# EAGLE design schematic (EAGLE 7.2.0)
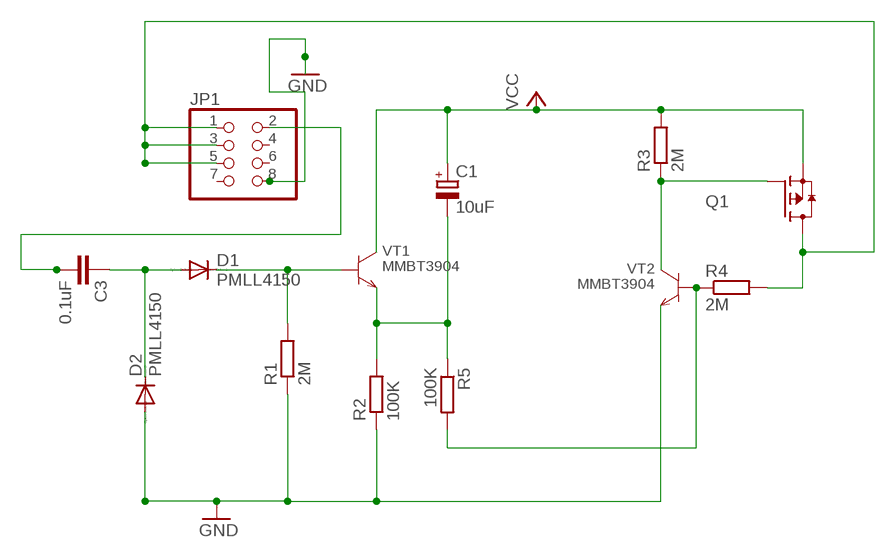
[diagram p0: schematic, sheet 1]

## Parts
C1  10uF  CPOL-EU153CLV-0505  [153CLV-0505]
C3  0.1uF  C-EUC0805  [C0805]
D1  PMLL4150  [SOD80C]
D2  PMLL4150  [SOD80C]
JP1  PINHD-2X4  [2X04]
Q1  BSS84  [SOT-23]
R1  2M  R-EU_R0805  [R0805]
R2  100K  R-EU_R0805  [R0805]
R3  2M  R-EU_R0805  [R0805]
R4  2M  R-EU_R0805  [R0805]
R5  100K  R-EU_R0805  [R0805]
VT1  MMBT3904  [SOT23-BEC]
VT2  MMBT3904  [SOT23-BEC]

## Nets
GND: D2.A JP1.8 R1.1 R2.1 VT2.E
N$1: C3.2 JP1.2
N$2: D1.C R1.2 VT1.B
N$4: C1.- R2.2 R5.1 VT1.E
N$5: JP1.1 JP1.3 JP1.5 Q1.3(D) R4.2
N$6: R4.1 R5.2 VT2.B
N$7: Q1.1(G) R3.1 VT2.C
N$8: C3.1 D1.A D2.C
VCC: C1.+ Q1.2(S) R3.2 VT1.C
Unconnected: JP1.4 JP1.6 JP1.7

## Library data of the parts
C1 = rcl:CPOL-EU: POLARIZED CAPACITOR, European symbol
C3 = rcl:C-EU: CAPACITOR, European symbol
D1 D2 = diode:PMLL4150: DIODE
JP1 = pinhead:PINHD-2X4: PIN HEADER
Q1 = AWJLEagleLib:BSS84: BSS84 P-channel MOSFET
R1-R5 = rcl:R-EU_: RESISTOR, European symbol
VT1 VT2 = transistor-npn:MMBT3904*: NPN TRANSISTOR

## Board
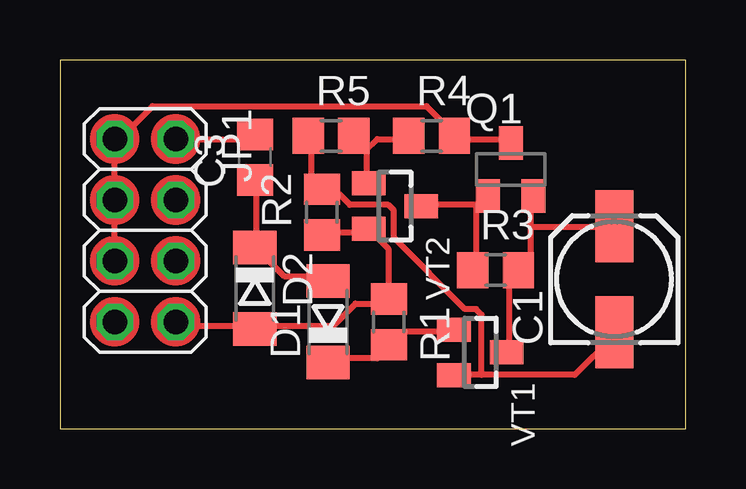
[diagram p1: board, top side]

Size 26.09 x 15.36 mm. Coordinates in mm from the lower left corner, seen from the top.
Outline: 0,0 26.09,0 26.09,15.36 0,15.36 0,0
Copper layers (1*16): Top 0.035mm / dielectric 1.5mm / Bottom 0.035mm
Design rules "default": minimum track width 10mil, minimum drill 24mil, track to track 8mil, track to pad 8mil, pad to pad 8mil, via to via 8mil, smd to smd 8mil, copper to edge 40mil, drill to drill 8mil, minimum pad ring 10mil, minimum via ring 8mil, stop-mask expansion 4mil, vias tented up to drill 0mil, thermal gap 10mil

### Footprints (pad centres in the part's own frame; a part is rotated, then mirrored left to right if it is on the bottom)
153CLV-0505 = smd 3 x 1.6: + 2.2,0; - -2.2,0
C0805 = smd 1.3 x 1.5: 1 -0.95,0; 2 0.95,0
SOD80C = smd 1.4 x 1.8: A 1.7,0; C -1.7,0
2X04 = drill 1.016 octagon: 1 -3.81,-1.27; 2 -3.81,1.27; 3 -1.27,-1.27; 4 -1.27,1.27; 5 1.27,-1.27; 6 1.27,1.27; 7 3.81,-1.27; 8 3.81,1.27
SOT-23 = smd 1 x 1.4: 1 -0.95,-1.1; 2 0.95,-1.1; 3 0,1.1
R0805 = smd 1.3 x 1.5: 1 -0.95,0; 2 0.95,0
SOT23-BEC = smd 1 x 1.4: B -0.95,-1.1; C 0,1.1; E 0.95,-1.1

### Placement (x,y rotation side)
C1  23.11,6.22 90 top
C3  8.13,11.3 90 top
D1  11.18,4.45 90 top
D2  8.13,5.84 270 top
JP1  3.56,8.26 270 top
Q1  18.8,10.8 0 top
R1  13.72,4.45 270 top
R2  10.92,9.02 90 top
R3  18.16,6.6 0 top
R4  15.49,12.19 0 top
R5  11.3,12.19 0 top
VT1  17.53,3.17 270 top
VT2  13.97,9.27 270 top

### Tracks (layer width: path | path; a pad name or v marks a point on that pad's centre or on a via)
GND
  Top 0.254: R2.1 10.95,8.18 12.78,8.18 VT2.E 13.01,8.18 13.69,7.49 13.69,5.44 R1.1 13.69,5.21 12.32,5.21 11.41,4.29 8.2,4.29 D2.A 7.98,4.29 5,4.29 JP1.8
N$1
  Top 0.254: JP1.2 7.98,12.06 C3.2
N$2
  Top 0.254: VT1.B 16.2,4.06 14.38,4.06 13.92,3.61 R1.2 13.69,3.38 13.23,2.92 11.18,2.92 D1.C
N$4
  Top 0.254: R5.1 10.49,12.06 10.49,10.24 10.72,10.01 R2.2 10.95,9.78 11.63,9.78 12.09,9.32 13.69,9.32 13.92,9.09 13.92,7.95 16.89,4.98 17.35,4.98 17.58,4.75 17.58,2.23 | 17.58,2.23 21.46,2.23 23.06,3.84 C1.- | 17.58,2.23 VT1.E
N$5
  Top 0.254: Q1.3 18.72,12.06 16.66,12.06 R4.2 16.43,12.29 15.29,13.44 3.86,13.44 2.49,12.06 JP1.1 JP1.3 JP1.5
N$6
  Top 0.254: 12.78,11.61 12.78,10.24 VT2.B | 12.78,11.61 12.32,12.06 R5.2 12.78,11.61 | 12.78,11.61 13.23,12.06 14.38,12.06 R4.1
N$7
  Top 0.254: 17.35,9.32 17.58,9.32 17.8,9.55 Q1.1 17.35,9.32 | 17.35,9.32 15.29,9.32 VT2.C | 17.35,9.32 17.35,6.81 R3.1
N$8
  Top 0.254: C3.1 8.2,10.24 8.2,7.72 D2.C 8.2,7.49 9.35,6.35 11.18,6.35 D1.A
VCC
  Top 0.254: VT1.C 18.72,3.38 18.72,6.35 18.95,6.58 R3.2 19.18,6.81 19.63,7.26 19.63,8.41 | 19.63,8.41 19.63,9.55 Q1.2 | 19.63,8.41 23.06,8.41 C1.+
(copper drawn outside any net)
  shapes: Top circle x8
